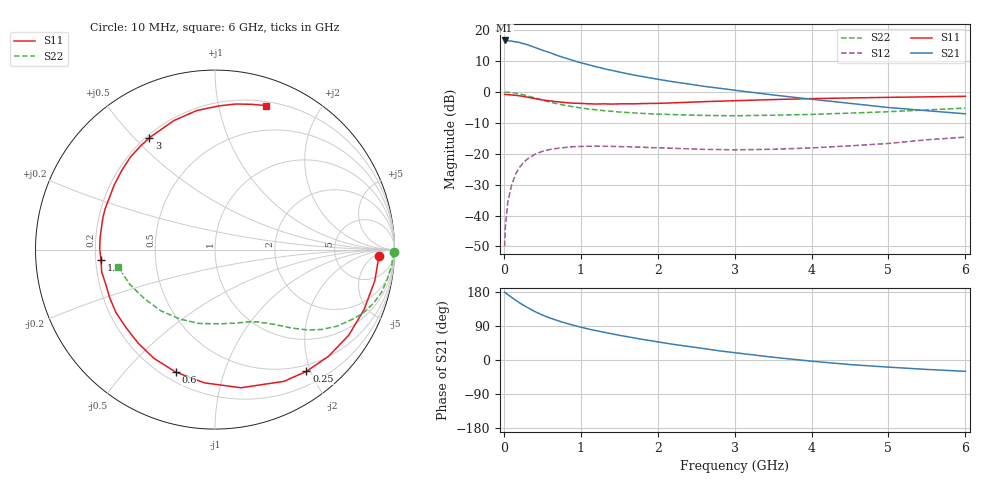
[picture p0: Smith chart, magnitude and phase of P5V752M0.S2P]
! SIEMENS Small Signal Semiconductors
! BFP183
! Si NPN RF Bipolar Junction Transistor in SOT143
! VCE = 0.75 V  IC = 2 mA
! Common Emitter S-Parameters:  March  1996
# GHz  S  MA  R  50
!  f  S11  S21  S12  S22
! GHz  MAG  ANG  MAG  ANG  MAG  ANG  MAG  ANG
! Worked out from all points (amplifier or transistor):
!   36 points, 10 MHz to 6 GHz, reference 50 ohm
!   highest |S21| = 16.7 dB at 10 MHz (marker M1)
!   |S21| within 3 dB of that: start of sweep to 483.8 MHz
!   unconditionally stable (mu >= 1): 1.976 GHz to end of sweep
!   at 250 MHz: K = 0.13, MSG = 19.3 dB, |S12| = -23.0 dB
!   at 1.4 GHz: K = 0.71, MSG = 12.3 dB, |S12| = -17.6 dB
!   at 6 GHz: K = 1.13, MAG = 1.6 dB, |S12| = -14.6 dB
!   S11 on the Smith chart (normalised r, x): 10 MHz: 19, -8; 250 MHz: 0.40, -1.94; 600 MHz: 0.25, -0.70; 1.4 GHz: 0.22, -0.04; 3 GHz: 0.21, +0.55; 6 GHz: 0.24, +1.39
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0.01  0.9154 -2.1  6.825 178.9  0.0032 89.4  0.9979 -0.9
0.02  0.9101 -4.6  6.81 177.6  0.0066 88.0  0.9902 -2.0
0.05  0.907 -11.1  6.777 172.7  0.0161 84.6  0.9893 -4.9
0.1  0.8951 -22.0  6.655 165.5  0.0309 77.6  0.9738 -9.7
0.2  0.8683 -43.1  6.333 151.5  0.0594 65.7  0.9322 -18.7
0.25  0.8484 -53.1  6.091 145.0  0.0709 60.1  0.901 -22.8
0.3  0.8288 -62.3  5.856 139.4  0.0813 55.5  0.8661 -26.2
0.4  0.7834 -79.3  5.284 128.1  0.0977 46.9  0.803 -32.1
0.5  0.7447 -94.6  4.749 118.7  0.1095 39.6  0.7412 -36.9
0.6  0.7168 -107.7  4.324 110.8  0.1176 33.5  0.6873 -40.7
0.7  0.6949 -119.4  3.879 103.9  0.1228 28.8  0.6418 -43.5
0.8  0.6743 -129.5  3.544 97.6  0.1267 24.7  0.6062 -46.0
0.9  0.6594 -138.7  3.239 92.0  0.1302 21.2  0.5776 -47.9
1.1  0.6452 -155.4  2.765 81.7  0.1325 15.7  0.5307 -51.6
1.4  0.6377 -175.0  2.239 69.3  0.1319 9.5  0.4873 -56.8
1.8  0.6496 164.0  1.78 54.5  0.1278 5.5  0.4506 -63.0
2.2  0.667 147.3  1.463 41.4  0.1229 3.3  0.4312 -70.7
3  0.7226 120.4  1.069 19.3  0.1159 5.2  0.413 -89.2
3.5  0.7544 107.7  0.896 7.3  0.1184 8.6  0.4211 -102.0
4.5  0.8008 88.5  0.655 -12.1  0.1345 13.6  0.4558 -131.7
5.5  0.8346 75.9  0.498 -24.9  0.1689 14.4  0.5136 -158.1
6  0.8518 70.4  0.444 -29.9  0.186 11.4  0.5477 -170.0
